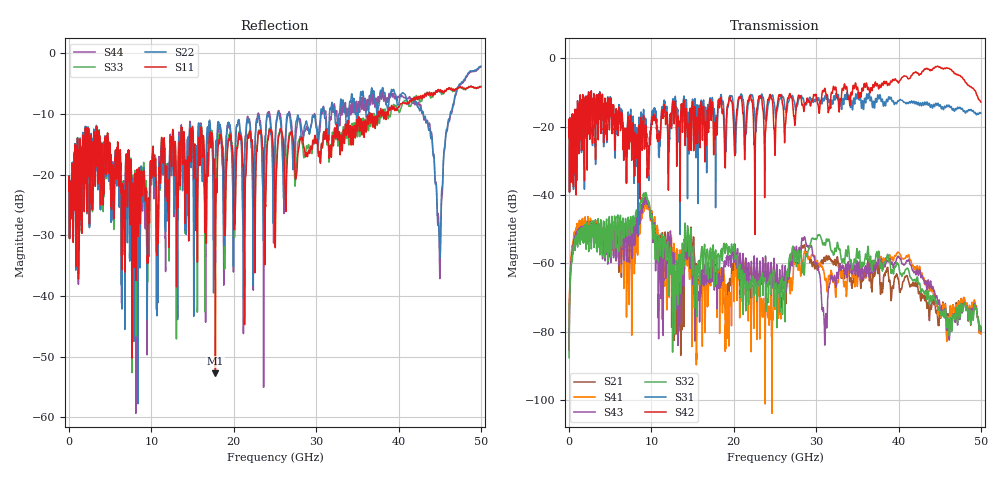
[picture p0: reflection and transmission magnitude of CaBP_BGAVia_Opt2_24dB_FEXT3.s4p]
!* Samtec Inc. NovaRay Examax Flyover System  *
!*  REV DATE  = 08/08/18  *
!*  TYPE  = TOUCHSTONE  *
!*  PORTS  = 4 port  *
!*  UNITS  = GHz  *
!*  DATA RANGE = DC  to 50 GHz; 10 MHz Step  *
!*  PARAMETER  = S  *
!*  FORMAT  = Real-Imaginary  *
!*  REFERENCE  = 50 ohms  *
!*  SOURCE  = HFSS  *
!*  VALIDATED  = No  *
!*  MANUFACTURER = SAMTEC  *
!*  INTERCONNECT = NVAx to EBCx to EBCx to NVAx  *
!*  [Full Channel NVAx to EBCx to EBCx to NVAx  with PCB Trace and BGA Via]  *
!*  BOUNDARY A  = Silicon BGA Ball Pad  *
!*  BOUNDARY B  = Silicon BGA Ball Pad  *
!*  NVAx (end a) ->>- (end b) NVAx  *
!*  Port 01 ->>- Port 02  *
!*  Port 03 ->>- Port 04  *
!***************************** CHANNEL MODEL ******************************************
# GHz S RI R 50
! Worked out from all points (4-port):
!   5000 points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, 10 MHz to 50 GHz, reference 50 ohm
!   strongest paths, dB at 10 MHz, 12.51 GHz, 25.01 GHz, 37.51 GHz, 50 GHz:
!     S42: -23.2, -14.9, -28.2, -8.0, -12.8
!     S31: -23.2, -14.5, -15.2, -10.7, -16.0
!     S32: -87.6, -69.2, -66.3, -58.3, -79.6
!     S43: -85.6, -58.0, -66.5, -59.8, -79.9
!     S41: -83.4, -56.9, -71.3, -59.3, -80.7
!     S21: -85.0, -62.5, -66.2, -62.9, -80.2
!   lowest |S11| = -52.7 dB at 17.77 GHz (marker M1), VSWR 1.00, Z = 49.8 - j0.145 ohm
!   |S11| at or under -10 dB: start of sweep to 36.46 GHz; 36.55 GHz to 36.75 GHz (204 MHz wide, 0.557 % of centre); 36.79 GHz to 37.51 GHz (722.9 MHz wide, 1.95 % of centre)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
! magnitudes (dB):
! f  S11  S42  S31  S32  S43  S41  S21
! 10 MHz  -22.7  -23.2  -23.2  -87.6  -85.6  -83.4  -85.0
! 9.24 GHz  -22.9  -23.3  -20.4  -40.0  -41.2  -41.6  -40.6
! 13.19 GHz  -24.1  -17.4  -15.1  -64.6  -66.0  -58.7  -73.2
! 17.77 GHz  -52.7  -22.7  -28.1  -56.7  -65.5  -61.3  -62.1
! 39.31 GHz  -9.2  -6.2  -12.5  -62.4  -60.7  -58.9  -66.8
! 44.94 GHz  -6.3  -2.6  -14.0  -72.9  -70.7  -73.9  -76.8
! 50 GHz  -5.5  -12.8  -16.0  -79.6  -79.9  -80.7  -80.2
